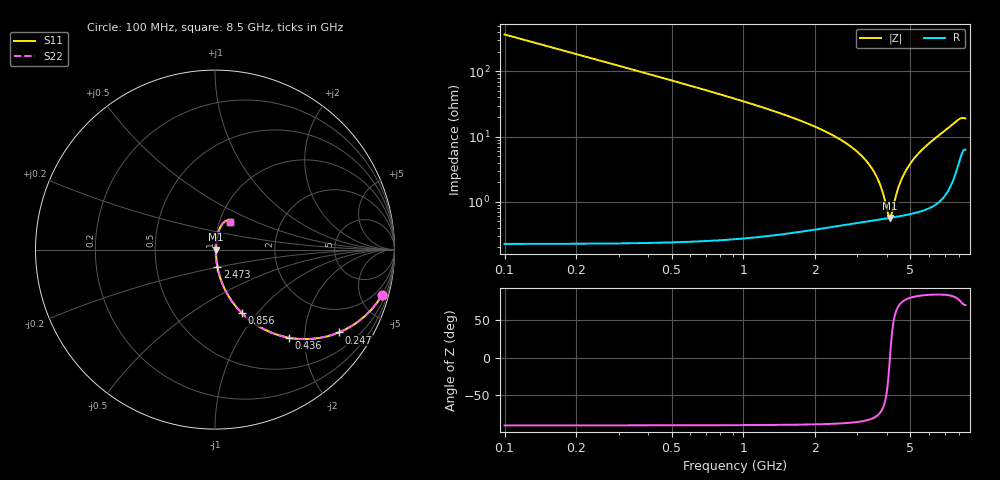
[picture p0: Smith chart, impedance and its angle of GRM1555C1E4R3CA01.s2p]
!Murata Part Number: GRM1555C1E4R3CA01
!These Parameters are Measured in Series Mode Connection
!  o--ll--o
!Port1  Port2
!  o------o
!Operation Temp=25[C], DC Bias Voltage=0[V]
!Freq. Start=100[MHz] Stop=8500[MHz] 401[Steps]
# Hz S RI R 50
!Freq.(Hz) S11(Real) S11(Imag) S21(Real) S21(Imag) S12(Real) S12(Imag) S22(Real) S22(Imag)
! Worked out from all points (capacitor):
!   401 points, 100 MHz to 8.5 GHz, reference 50 ohm
!   read as one part in series: C = 4.3 pF near 142 MHz
!   lowest |Z| = 567 mohm at 4.111 GHz (marker M1)
!   series resonance near 4.105 GHz, so ESL is about 350 pH
!   S11 on the Smith chart (normalised r, x): 100 MHz: 1.00, -7.40; 247 MHz: 1.00, -2.99; 436 MHz: 1.00, -1.68; 856 MHz: 1.01, -0.83; 2.473 GHz: 1.01, -0.19; 8.5 GHz: 1.13, +0.36
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1e8  0.9318 -0.2518  0.0682 0.2518  0.0682 0.2518  0.9318 -0.2518
2.47e8  0.6901 -0.4617  0.3099 0.4617  0.3099 0.4617  0.6901 -0.4617
4.36e8  0.4135 -0.4911  0.5865 0.4911  0.5865 0.4911  0.4135 -0.4911
6.25e8  0.2516 -0.4318  0.7484 0.4318  0.7484 0.4318  0.2516 -0.4318
8.56e8  0.1477 -0.3516  0.8523 0.3516  0.8523 0.3516  0.1477 -0.3516
1.507e9  0.0461 -0.2023  0.9539 0.2023  0.9539 0.2023  0.0461 -0.2023
2.473e9  0.0132 -0.0943  0.9868 0.0943  0.9868 0.0943  0.0132 -0.0943
2.914e9  0.00862 -0.0629  0.9914 0.0629  0.9914 0.0629  0.00862 -0.0629
3.313e9  0.00653 -0.0392  0.9935 0.0392  0.9935 0.0392  0.00653 -0.0392
3.607e9  0.00579 -0.0237  0.9942 0.0237  0.9942 0.0237  0.00579 -0.0237
3.817e9  0.00558 -0.0134  0.9944 0.0134  0.9944 0.0134  0.00558 -0.0134
4.048e9  0.00559 -0.0026  0.9944 0.0026  0.9944 0.0026  0.00559 -0.0026
4.111e9  0.00564 0.00025  0.9944 -0.00025  0.9944 -0.00025  0.00564 0.00025
4.174e9  0.0057 0.00307  0.9943 -0.00307  0.9943 -0.00307  0.0057 0.00307
4.3e9  0.00587 0.0086  0.9941 -0.0086  0.9941 -0.0086  0.00587 0.0086
4.51e9  0.00628 0.0176  0.9937 -0.0176  0.9937 -0.0176  0.00628 0.0176
4.804e9  0.00713 0.0298  0.9929 -0.0298  0.9929 -0.0298  0.00713 0.0298
5.203e9  0.00876 0.0458  0.9912 -0.0458  0.9912 -0.0458  0.00876 0.0458
5.707e9  0.0117 0.0656  0.9883 -0.0656  0.9883 -0.0656  0.0117 0.0656
7.114e9  0.0296 0.1249  0.9704 -0.1249  0.9704 -0.1249  0.0296 0.1249
7.996e9  0.0668 0.1618  0.9332 -0.1618  0.9332 -0.1618  0.0668 0.1618
8.5e9  0.0853 0.1544  0.9147 -0.1544  0.9147 -0.1544  0.0853 0.1544
